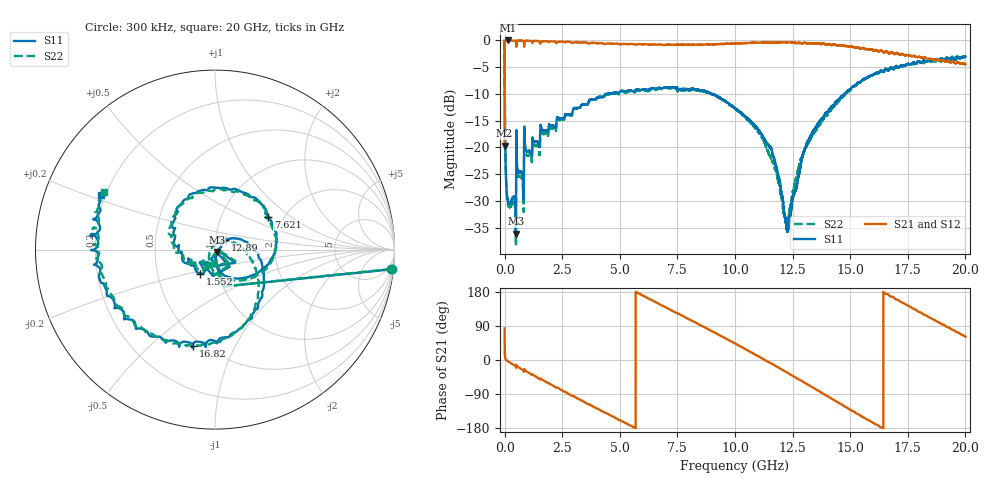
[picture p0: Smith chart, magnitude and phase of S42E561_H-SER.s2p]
! Created Wed Nov 25 22:21:33 2020
# khz S ma R 50
! 2 Port Network Data from SP1.SP block
! freq  magS11  angS11  magS21  angS21  magS12  angS12  magS22  angS22
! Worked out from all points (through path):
!   20001 points, 300 kHz to 20 GHz, reference 50 ohm
!   highest |S21| = -0.05 dB at 157.3 MHz (marker M1); lowest = -19.7 dB at 300 kHz (marker M2)
!   group delay of S21, straight-line fit = 91.8 ps
!   lowest |S11| = -36.1 dB at 490.3 MHz (marker M3), VSWR 1.03, Z = 50.9 - j1.29 ohm
!   |S11| at or under -10 dB: 8.616 MHz to 4.401 GHz (4.392 GHz wide, 199 % of centre); 4.561 GHz to 4.617 GHz (55.89 MHz wide, 1.22 % of centre); 8.989 GHz to 14.76 GHz (5.774 GHz wide, 48.6 % of centre)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
!   |S22| runs from -38.4 to -0.1 dB; largest |S21 - S12| = 0.017
!   S11 on the Smith chart (normalised r, x): 300 kHz: 2, -18; 1.552 GHz: 0.82, -0.23; 7.621 GHz: 1.67, +0.69; 12.89 GHz: 1.11, +0.12; 16.82 GHz: 0.45, -0.69; 20 GHz: 0.18, +0.22
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300  0.9895 -6.4  0.104 83.4  0.1037 83.2  0.9903 -6.2
101300  0.03627 -83.8  0.9929 -1.7  0.9939 -1.8  0.03554 -83.5
157300  0.03023 -85.5  0.9946 -4.2  0.9944 -4.2  0.02907 -84.5
490300  0.01568 -54.1  0.9857 -17.9  0.9856 -17.9  0.01199 -40.1
939300  0.09357 -118.7  0.9863 -29.6  0.987 -29.7  0.08584 -117.8
1552300  0.1585 -121.0  0.9341 -48.9  0.9338 -49.0  0.1399 -122.5
3334300  0.2484 158.8  0.948 -106.6  0.9483 -106.6  0.2468 169.5
5184300  0.3349 109.9  0.9237 -164.2  0.9233 -164.3  0.3292 105.5
6667300  0.3584 60.8  0.9099 149.2  0.9092 149.1  0.3507 59.0
7621300  0.349 31.4  0.9042 119.8  0.9065 119.8  0.3407 28.6
8803300  0.3287 -4.8  0.9129 82.4  0.9108 82.2  0.326 -9.8
1.00003e7  0.2331 -42.0  0.933 43.6  0.9321 43.6  0.2297 -47.7
1.15503e7  0.0991 -82.9  0.9461 -8.3  0.9441 -8.3  0.08146 -108.1
1.22593e7  0.01739 -30.6  0.9544 -33.3  0.9537 -33.3  0.02104 135.2
1.28943e7  0.07713 43.5  0.9368 -55.2  0.9386 -55.4  0.07957 39.7
1.33343e7  0.1326 27.1  0.9385 -71.0  0.9372 -71.2  0.1279 13.6
1.43203e7  0.2557 -11.9  0.9114 -106.5  0.9088 -106.4  0.2466 -24.1
1.52763e7  0.3889 -52.0  0.8568 -141.3  0.8593 -141.2  0.3858 -54.4
1.66673e7  0.522 -100.2  0.7591 172.1  0.7636 171.3  0.54 -98.2
1.68183e7  0.5497 -103.0  0.7728 166.8  0.7617 166.8  0.5463 -103.0
1.83943e7  0.6504 -156.6  0.6728 113.7  0.679 113.4  0.6267 -153.8
2e7  0.7034 154.5  0.5991 61.5  0.599 61.9  0.7039 152.5
